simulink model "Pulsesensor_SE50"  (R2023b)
settings: Solver=FixedStepDiscrete  StartTime=0.0  StopTime=inf  FixedStep=0.003  RelTol=1e-3  EnableMultiTasking=on
libraries: arduinolib x10

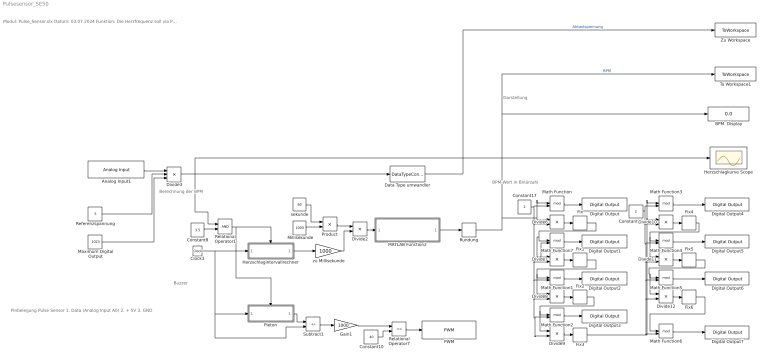
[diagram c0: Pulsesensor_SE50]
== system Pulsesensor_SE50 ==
  note: Darstellung
  note: Berechnung der BPM
  note: Buzzer
  note: BPM-Wert in Binärzahl
  note: Pinbelegung Pulse Sensor 1. Data (Analog Input A0) 2. + 5V 3. GND
  note: Modul: Pulse_Sensor.slx Datum: 03.07.2024 Funktion: Die Herzfrequenz soll via Pulse-Sensor in bpm gemessen werden. Implementierung: Simulink R2023b Toolbox: Simulink Support Package for Arduino Hardware Autor: Weiran Wang Letzte Änderung: 27.07.2024
  " Millisekunde" : Constant  Value=1000
  Analog Input1 : arduinolib/Analog Input  pinNumber=0  ReadResultsOnly=off  ConversionTriggerSource=Software  ExternalTriggerType=uint32( 0 )  OutputDataType=uint16  EnableConversionCompleteNotify=off  EnableOuputStatus=off  SampleTime=-1  blockPlatform=arduino
  BPM  Display : Display
  Clock3 : Clock
  Constant10 : Constant  Value=40
  Constant17 : Constant  Value=2
  Constant18 : Constant  Value=2
  Constant8 : Constant  Value=3.5
  Data Type umwandler : DataTypeConversion  OutDataTypeStr=double
  Digital Output : arduinolib/Digital Output  pinNumber=6  Direction=output  blockPlatform=arduino
  Digital Output1 : arduinolib/Digital Output  pinNumber=7  Direction=output  blockPlatform=arduino
  Digital Output2 : arduinolib/Digital Output  pinNumber=8  Direction=output  blockPlatform=arduino
  Digital Output3 : arduinolib/Digital Output  pinNumber=9  Direction=output  blockPlatform=arduino
  Digital Output4 : arduinolib/Digital Output  pinNumber=10  Direction=output  blockPlatform=arduino
  Digital Output5 : arduinolib/Digital Output  pinNumber=11  Direction=output  blockPlatform=arduino
  Digital Output6 : arduinolib/Digital Output  pinNumber=12  Direction=output  blockPlatform=arduino
  Digital Output7 : arduinolib/Digital Output  pinNumber=13  Direction=output  blockPlatform=arduino
  Divide{2,6..12} (8 alike) : Product  Inputs=*/
  Divide3 : Product  Inputs=**/
  Fix{,1..6} (7 alike) : Rounding  Operator=fix
  Gain1 : Gain  Gain=1000
  Herzschlagintervallrechner : Subsystem  TreatAsAtomicUnit=on
  Herzschlagkurve Scope : Scope
  MATLAB Function2 : MATLAB Function  TreatAsAtomicUnit=on
  Math Function{,1..7} (8 alike) : Math  Operator=mod
  Maximum Digital Output : Constant  Value=1023
  PWM : arduinolib/PWM  pinNumber=5  frequencyType=Default  desiredFrequency=490.2  achievableFrequency=490.2
  Pieton : Subsystem  TreatAsAtomicUnit=on
  Product : Product
  Referenzspannung : Constant  Value=5
  Relational Operator1 : RelationalOperator  OutDataTypeStr=boolean  RndMeth=Simplest
  Relational Operator7 : RelationalOperator  Operator=<=  OutDataTypeStr=boolean  RndMeth=Simplest
  Rundung : Rounding
  Subtract1 : Sum  Inputs=-+
  To Workspace1 : ToWorkspace  VariableName=simout1  SampleTime=-1
  Zu Workspace : ToWorkspace  VariableName=simout  SampleTime=-1
  sekunde : Constant  Value=60
  zu Millisekunde : Gain  Gain=1000
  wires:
  Divide3/1 -> Relational Operator1/1, Herzschlagkurve Scope/1, Data Type umwandler/1
  Constant8/1 -> Relational Operator1/2
  Relational Operator1/1 -> Pieton/Trigger, Herzschlagintervallrechner/Trigger
  Herzschlagintervallrechner/1(Out1) -> zu Millisekunde/1
  sekunde/1 -> Product/1
  " Millisekunde"/1 -> Product/2
  Product/1 -> Divide2/1
  zu Millisekunde/1 -> Divide2/2
  Data Type umwandler/1 -> Zu Workspace/1  "Abtastspannung"
  Analog Input1/1 -> Divide3/1
  Referenzspannung/1 -> Divide3/2
  Maximum Digital Output/1 -> Divide3/3
  Divide2/1 -> MATLAB Function2/1(BPM)
  Rundung/1 -> To Workspace1/1, BPM  Display/1, Math Function/1, Divide6/1  "BPM"
  MATLAB Function2/1(BPM_Median) -> Rundung/1
  Pieton/1(Outport) -> Subtract1/1
  Clock3/1 -> Subtract1/2, Pieton/1(Input), Herzschlagintervallrechner/1(In1)
  Subtract1/1 -> Gain1/1
  Gain1/1 -> Relational Operator7/1
  Constant10/1 -> Relational Operator7/2
  Relational Operator7/1 -> PWM/1
  Math Function/1 -> Digital Output/1
  Divide6/1 -> Fix/1
  Fix/1 -> Divide7/1, Math Function7/1
  Math Function7/1 -> Digital Output1/1
  Divide7/1 -> Fix1/1
  Fix1/1 -> Divide8/1, Math Function1/1
  Constant17/1 -> Divide9/2, Math Function2/2, Divide8/2, Math Function1/2, Divide7/2, Math Function7/2, Divide6/2, Math Function/2
  Divide8/1 -> Fix2/1
  Math Function1/1 -> Digital Output2/1
  Fix2/1 -> Math Function2/1, Divide9/1
  Math Function2/1 -> Digital Output3/1
  Constant18/1 -> Math Function3/2, Divide10/2, Math Function6/2, Divide12/2, Math Function5/2, Divide11/2, Math Function4/2
  Divide9/1 -> Fix3/1
  Math Function3/1 -> Digital Output4/1
  Fix3/1 -> Divide10/1, Math Function3/1
  Divide10/1 -> Fix4/1
  Divide11/1 -> Fix5/1
  Divide12/1 -> Fix6/1
  Math Function4/1 -> Digital Output5/1
  Fix4/1 -> Divide11/1, Math Function4/1
  Fix5/1 -> Divide12/1, Math Function5/1
  Math Function5/1 -> Digital Output6/1
  Fix6/1 -> Math Function6/1
  Math Function6/1 -> Digital Output7/1

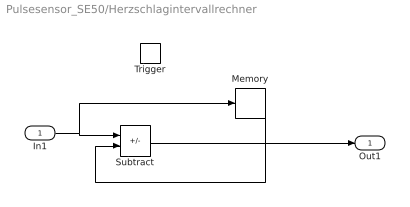
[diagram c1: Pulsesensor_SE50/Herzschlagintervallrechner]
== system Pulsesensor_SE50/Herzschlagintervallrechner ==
  In1 : Inport
  Trigger : TriggerPort  VariantControl=(inherit)
  Memory : Memory  InheritSampleTime=on
  Subtract : Sum  Inputs=+-
  Out1 : Outport
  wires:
  In1/1 -> Memory/1, Subtract/1
  Subtract/1 -> Out1/1
  Memory/1 -> Subtract/2

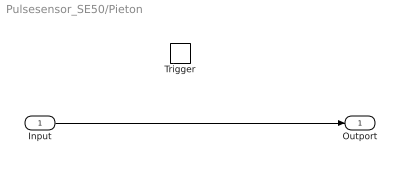
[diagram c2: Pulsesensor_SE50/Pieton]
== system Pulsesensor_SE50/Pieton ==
  Input : Inport
  Trigger : TriggerPort  VariantControl=(inherit)
  Outport : Outport
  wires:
  Input/1 -> Outport/1

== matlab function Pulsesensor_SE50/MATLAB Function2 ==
function BPM_Median = Medianfilter(BPM)

persistent bInit aSchieberegister n 
if isempty(bInit)
   bInit=1;
   n = 15;
   aSchieberegister = ones(1,n)*BPM;
end

aSchieberegister(1:end-1)=aSchieberegister(2:end);
aSchieberegister(end)=BPM;

aSortiertesRegister = sort(aSchieberegister);

BPM_Median = aSortiertesRegister(ceil(n/2));

end
